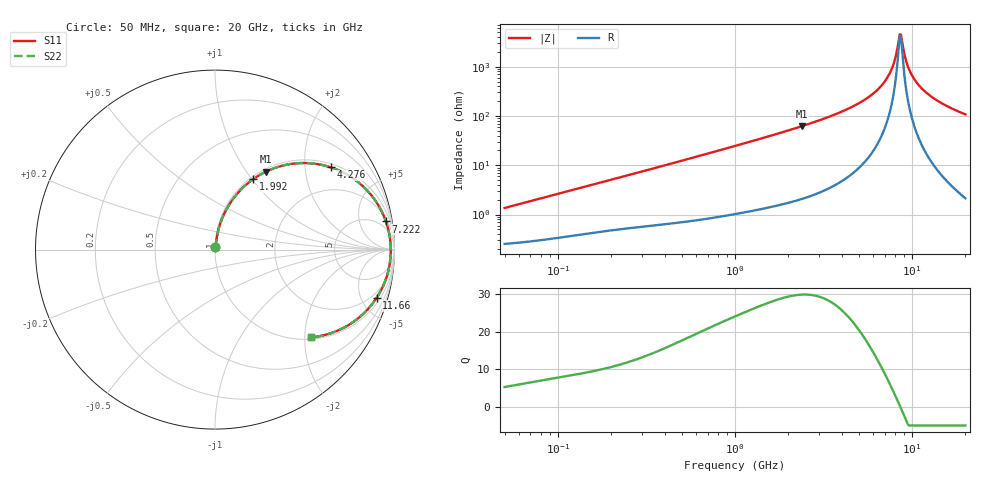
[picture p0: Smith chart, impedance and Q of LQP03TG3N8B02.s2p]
!Murata Part Number: LQP03TG3N8B02
!These Parameters are Measured in Series Mode Connection
!  o--[Z]--o
!Port1  Port2
!  o-------o
!Freq. Start=50[MHz] Stop=20[GHz], 401[Steps]
# Hz S RI R 50
!Freq.(Hz) S11(Real) S11(Imag) S21(Real) S21(Imag) S12(Real) S12(Imag) S22(Real) S22(Imag)
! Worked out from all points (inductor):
!   401 points, 50 MHz to 20 GHz, reference 50 ohm
!   read as one part in series: L = 4.24 nH near 51.52 MHz
!   highest Q = 30 at 2.384 GHz (marker M1), where L = 4.14 nH
!   self-resonance near 8.516 GHz
!   S11 on the Smith chart (normalised r, x): 50 MHz: 1.01, +0.03; 1.992 GHz: 1.03, +1.01; 4.276 GHz: 1.11, +2.72; 7.222 GHz: 3, +12; 11.66 GHz: 1.42, -6.54; 20 GHz: 1.04, -2.15
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5e7  0.00271 0.0133  0.9973 -0.0133  0.9973 -0.0133  0.00271 0.0133
1.364002e8  0.00517 0.0349  0.9948 -0.0349  0.9948 -0.0349  0.00517 0.0349
3.721004e8  0.0145 0.0905  0.9855 -0.0905  0.9855 -0.0905  0.0145 0.0905
1e9  0.0657 0.2278  0.9343 -0.2278  0.9343 -0.2278  0.0657 0.2278
1.99176e9  0.2122 0.3922  0.7878 -0.3922  0.7878 -0.3922  0.2122 0.3922
2.383959e9  0.2845 0.4348  0.7155 -0.4348  0.7155 -0.4348  0.2845 0.4348
2.728004e9  0.3513 0.4609  0.6487 -0.4609  0.6487 -0.4609  0.3513 0.4609
4.275624e9  0.6439 0.4589  0.3561 -0.4589  0.3561 -0.4589  0.6439 0.4589
5.856089e9  0.8574 0.319  0.1426 -0.319  0.1426 -0.319  0.8574 0.319
6.601595e9  0.9189 0.232  0.0811 -0.232  0.0811 -0.232  0.9189 0.232
7.222371e9  0.9524 0.1571  0.0476 -0.1571  0.0476 -0.1571  0.9524 0.1571
7.442007e9  0.9607 0.1307  0.0393 -0.1307  0.0393 -0.1307  0.9607 0.1307
7.901521e9  0.9729 0.0764  0.0271 -0.0764  0.0271 -0.0764  0.9729 0.0764
8.389408e9  0.9789 0.0208  0.0211 -0.0208  0.0211 -0.0208  0.9789 0.0208
8.644534e9  0.9795 -0.00717  0.0205 0.00717  0.0205 0.00717  0.9795 -0.00717
8.774992e9  0.9791 -0.0212  0.0209 0.0212  0.0209 0.0212  0.9791 -0.0212
9.316812e9  0.9738 -0.0769  0.0262 0.0769  0.0262 0.0769  0.9738 -0.0769
9.745021e9  0.9657 -0.118  0.0343 0.118  0.0343 0.118  0.9657 -0.118
1.050288e10  0.9446 -0.184  0.0554 0.184  0.0554 0.184  0.9446 -0.184
1.166392e10  0.9006 -0.2689  0.0994 0.2689  0.0994 0.2689  0.9006 -0.2689
1.460232e10  0.7639 -0.4076  0.2361 0.4076  0.2361 0.4076  0.7639 -0.4076
2e10  0.5365 -0.4888  0.4635 0.4888  0.4635 0.4888  0.5365 -0.4888
